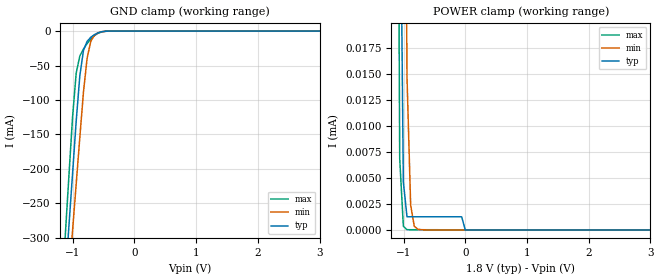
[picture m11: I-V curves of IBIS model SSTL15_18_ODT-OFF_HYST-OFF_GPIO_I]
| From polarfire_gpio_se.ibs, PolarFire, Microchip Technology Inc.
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|   Model SSTL15_18_ODT-OFF_HYST-OFF_GPIO_I
[Model]   SSTL15_18_ODT-OFF_HYST-OFF_GPIO_I
Model_type   Input
Vinl =   0.65
Vinh =   0.85
|   typ   min   max
C_comp_pullup   2.605e-12   2.605e-12   2.76e-12
C_comp_pulldown  2.605e-12   2.605e-12   2.76e-12
[Temperature Range]  25C   100C   -40C
[Voltage Range]  1.8   1.71   1.89
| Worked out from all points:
|   GND clamp passes 1 mA (typ) near -0.53 V on its own axis
[GND Clamp]
| Voltage   I(typ)   I(min)   I(max)
-1.8V     -1.238A    -1.206A    -1.294A
-1.122V   -360.2mA   -425.9mA   -297.3mA
-1.063V   -283.8mA   -358mA     -210.9mA
-1.004V   -207.4mA   -290mA     -125.4mA
-945mV    -131.1mA   -222.2mA   -61.15mA
-885.9mV  -64.84mA   -154.3mA   -36.15mA
-826.9mV  -28.05mA   -88.35mA   -26.02mA
-767.8mV  -14.97mA   -39.36mA   -18.12mA
-708.7mV  -9.067mA   -14.9mA    -11.6mA
-649.7mV  -5.157mA   -6.074mA   -6.592mA
-413.4mV  -46.15uA   -72.15uA   -56.26uA
3.6V      0A         0A         0A
[POWER Clamp]
| Voltage   I(typ)   I(min)   I(max)
-1.8V     692.2uA    1.143mA    803.1uA
-1.122V   247.5uA    167.5uA    79.37uA
-1.063V   40.35uA    140.6uA    6.852uA
-1.004V   4.6uA      75.51uA    361.6nA
-945mV    1.264uA    14.68uA    26.34nA
-885.9mV  1.264uA    2.392uA    22.42nA
-826.9mV  1.264uA    351.3nA    22.42nA
-767.8mV  1.264uA    67.95nA    22.42nA
-59.06mV  1.264uA    803.4pA    4.88nA
0V        0A         321.4pA    1.677nA
3.6V      0A         0A         0A
